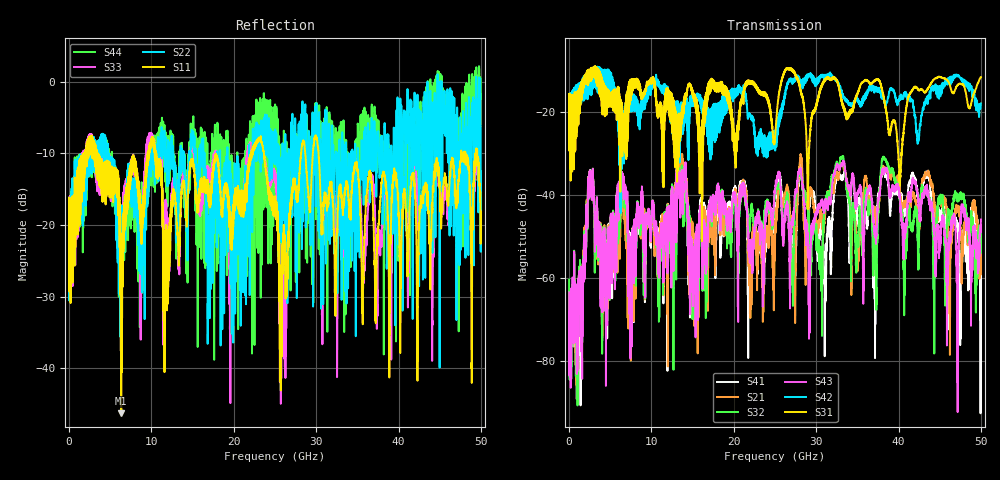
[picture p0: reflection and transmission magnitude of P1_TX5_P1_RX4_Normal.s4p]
!Keysight Technologies,N5225B,MY57041031,A.13.20.10
!Date: Friday, May 31, 2019 11:19:14
!Correction: S11(Full 4 Port(1,2,3,4))
!S12(Full 4 Port(1,2,3,4))
!S13(Full 4 Port(1,2,3,4))
!S14(Full 4 Port(1,2,3,4))
!S21(Full 4 Port(1,2,3,4))
!S22(Full 4 Port(1,2,3,4))
!S23(Full 4 Port(1,2,3,4))
!S24(Full 4 Port(1,2,3,4))
!S31(Full 4 Port(1,2,3,4))
!S32(Full 4 Port(1,2,3,4))
!S33(Full 4 Port(1,2,3,4))
!S34(Full 4 Port(1,2,3,4))
!S41(Full 4 Port(1,2,3,4))
!S42(Full 4 Port(1,2,3,4))
!S43(Full 4 Port(1,2,3,4))
!S44(Full 4 Port(1,2,3,4))
!S4P File: Measurements: <S11,S12,S13,S14>,
!<S21,S22,S23,S24>,
!<S31,S32,S33,S34>,
!<S41,S42,S43,S44>:
# Hz S  dB  R 50.0
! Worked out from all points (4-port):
!   5000 points, 10 MHz to 50 GHz, reference 50 ohm
!   strongest paths, dB at 10 MHz, 12.51 GHz, 25.01 GHz, 37.51 GHz, 50 GHz:
!     S31: -19.4, -23.0, -26.2, -12.3, -11.7
!     S42: -19.4, -19.4, -26.4, -14.8, -18.1
!     S43: -63.5, -39.6, -39.0, -41.8, -45.9
!     S32: -60.4, -38.7, -40.4, -44.9, -50.8
!     S21: -65.4, -42.2, -51.6, -45.4, -51.7
!     S41: -63.2, -43.8, -45.9, -40.0, -69.1
!   lowest |S11| = -46.3 dB at 6.34 GHz (marker M1), VSWR 1.01, Z = 49.6 - j0.262 ohm
!   |S11| at or under -10 dB: 3.502 GHz to 9.556 GHz (6.054 GHz wide, 92.7 % of centre); 10.5 GHz to 22.11 GHz (11.6 GHz wide, 71.2 % of centre); 30.29 GHz to 47.6 GHz (17.31 GHz wide, 44.4 % of centre)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
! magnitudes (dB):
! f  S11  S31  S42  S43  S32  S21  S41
! 10 MHz  -19.8  -19.4  -19.4  -63.5  -60.4  -65.4  -63.2
! 6.34 GHz  -46.3  -20.2  -23.9  -36.1  -37.8  -39.7  -37.6
! 30.57 GHz  -17.2  -14.1  -11.6  -42.1  -52.5  -44.3  -46.4
! 33.14 GHz  -17.1  -17.8  -15.4  -32.4  -31.0  -32.4  -36.0
! 37.08 GHz  -25.4  -12.6  -15.0  -48.5  -50.6  -43.3  -56.5
! 43.43 GHz  -14.3  -14.8  -16.5  -38.2  -39.0  -34.9  -35.1
! 50 GHz  -18.1  -11.7  -18.1  -45.9  -50.8  -51.7  -69.1
